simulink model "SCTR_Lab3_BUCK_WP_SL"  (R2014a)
settings: Solver=FixedStepDiscrete  StartTime=0.0  StopTime=2  FixedStep=1e-5  RelTol=1e-3
libraries: powerlib x12

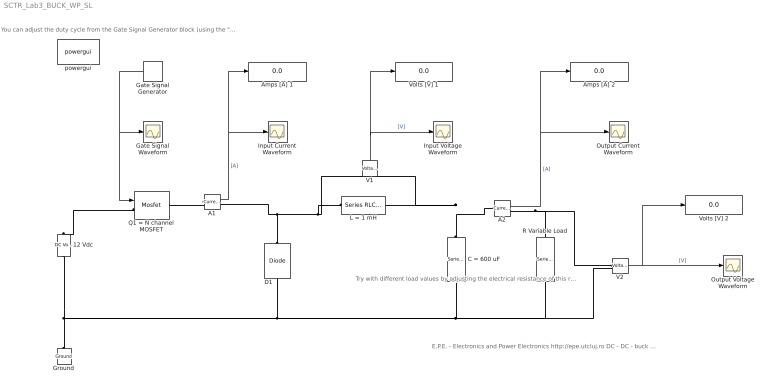
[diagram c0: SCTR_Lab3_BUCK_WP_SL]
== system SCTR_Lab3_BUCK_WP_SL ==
  note: E.P.E. - Electronics and Power Electronics http://epe.utcluj.ro DC - DC - buck converter - Simulink model Done by Pintilie Lucian Nicolae Lucian.Pintilie@emd.utcluj.ro
  note: Try with different load values by adjusting the electrical resistance of this resistor!
  note: You can adjust the duty cycle from the Gate Signal Generator block (using the "Pulse Width" parameter)!
  12 Vdc : powerlib/Electrical Sources/DC Voltage Source  Amplitude=12  Measurements=None
  A1 : powerlib/Measurements/Current Measurement  PhasorSimulation=off  OutputType=Complex  PSBequivalent=0
  A2 : powerlib/Measurements/Current Measurement  PhasorSimulation=off  OutputType=Complex  PSBequivalent=0
  Amps [A] 1 : Display
  Amps [A] 2 : Display
  C = 600 uF : powerlib/Elements/Series RLC Branch  LConnTagsString=__new0  RConnTagsString=__new0  BranchType=C  Resistance=1  Inductance=1e-3  SetiL0=off  InitialCurrent=0  Capacitance=600e-6  Setx0=on  InitialVoltage=0  Measurements=None
  D1 : powerlib/Power Electronics/Diode  Ron=0.001  Lon=0  Vf=0.8  IC=0  UseSnubber=off  Rs=500  Cs=250e-9  Measurements=off
  Gate Signal Waveform : Scope
  Gate Signal Generator : DiscretePulseGenerator  PulseType=Time based  Amplitude=15  Period=0.0001  PulseWidth=50
  Ground : powerlib/Elements/Ground  LConnTagsString=a
  Input Current Waveform : Scope
  Input Voltage Waveform : Scope
  L = 1 mH : powerlib/Elements/Series RLC Branch  LConnTagsString=__new0  RConnTagsString=__new0  BranchType=L  Resistance=1  Inductance=1e-3  SetiL0=off  InitialCurrent=0  Capacitance=1e-6  Setx0=off  InitialVoltage=0  Measurements=None
  Output Current Waveform : Scope
  Output Voltage Waveform : Scope
  Q1 = N channel MOSFET : powerlib/Power Electronics/Mosfet  Ron=0.1  Lon=0  Rd=0.01  Vfd=0  IC=0  Rs=1e5  Cs=inf  Measurements=off
  R Variable Load : powerlib/Elements/Series RLC Branch  LConnTagsString=__new0  RConnTagsString=__new0  BranchType=R  Resistance=10  Inductance=1e-3  SetiL0=off  InitialCurrent=0  Capacitance=800e-6  Setx0=on  InitialVoltage=0  Measurements=None
  V1 : powerlib/Measurements/Voltage Measurement  PhasorSimulation=off  OutputType=Complex  PSBequivalent=0
  V2 : powerlib/Measurements/Voltage Measurement  PhasorSimulation=off  OutputType=Complex  PSBequivalent=0
  Volts [V] 1 : Display
  Volts [V] 2 : Display
  powergui : powerlib/powergui  Priority=1  SimulationMode=Discrete  SolverType=Tustin  SampleTime=1e-5  frequency=60  SPID=off  DisableSnubberDevices=off  DisableRonSwitches=off  DisableVfSwitches=off  SwTol=0  DisplayEquations=off  Interpol=off  methode=off  Ts=0  FunctionMessages=off  echomessages=off  HookPort=off  EnableUseOfTLC=off  x0status=blocks  frequencyindice=0  Pbase=100e6  ErrMax=1e-4  Iterations=50  UnitsV=kV  UnitsW=MW  buscounter=0  RestoreLinks=warning  ResistiveCurrentMeasurement=off  Frange=[0:2:500]  Ylog=off  Xlog=on  ShowGrid=off  save=off  variable=ZData  structure=0  ZoomFFT=off  StartTime=0.0  cycles=1  DisplayStyle=1  fundamental=60  FreqAxis=off  MaxFrequency=1000  frequencyindicesteady=1  RmsSteady=1  display=off
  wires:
  V2/1 -> Output Voltage Waveform/1, Volts [V] 2/1  "[V]"
  A2/1 -> Amps [A] 2/1, Output Current Waveform/1  "[A]"
  V1/1 -> Volts [V] 1/1, Input Voltage Waveform/1  "[V]"
  Gate Signal Generator/1 -> Gate Signal Waveform/1, Q1 = N channel MOSFET/1
  A1/1 -> Input Current Waveform/1, Amps [A] 1/1  "[A]"
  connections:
  12 Vdc/LConn1 -- C = 600 uF/RConn1 -- R Variable Load/RConn1 -- V2/LConn2 -- D1/LConn1 -- Ground/LConn1
  A2/RConn1 -- R Variable Load/LConn1 -- V2/LConn1
  C = 600 uF/LConn1 -- L = 1 mH/RConn1 -- V1/LConn2 -- A2/LConn1
  D1/RConn1 -- L = 1 mH/LConn1 -- V1/LConn1 -- A1/RConn1
  Q1 = N channel MOSFET/LConn1 -- 12 Vdc/RConn1
  A1/LConn1 -- Q1 = N channel MOSFET/RConn1
